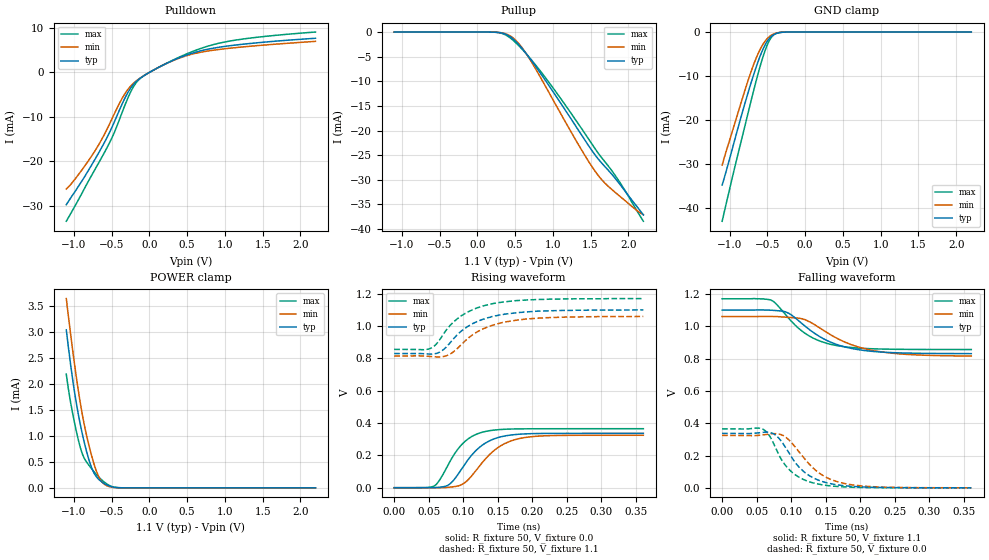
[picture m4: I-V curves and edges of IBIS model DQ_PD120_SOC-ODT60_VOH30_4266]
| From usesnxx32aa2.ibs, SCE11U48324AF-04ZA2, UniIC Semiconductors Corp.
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| DQ_PD120_SOC-ODT60_VOH30_4266
| (120 Ohm Pulldown, 60 Ohm System ODT Setting, VOH=VDDQ/3.0, 3200-4266Mbps)
[Model]   DQ_PD120_SOC-ODT60_VOH30_4266
Model_type   I/O
Vinl = 123.333mV
Vinh = 243.333mV
Vmeas = 183.333mV
Vref = 0.0mV
Cref = 0.0pF
Rref = 60.000Ohm
|   typ   min   max
|C_comp   0.797pF   0.747pF   0.847pF
C_comp_pullup   0.3985pF   0.3735pF   0.4235pF
C_comp_pulldown   0.3985pF   0.3735pF   0.4235pF
| Note: C_comp changes when the ODT circuit is enabled.
[Model Spec]
| Input threshold voltage corners
Vinl   0.1233V   0.1167V   0.1350V
Vinh   0.2433V   0.2367V   0.2550V
| Measurement voltage corners
Vmeas   0.1833V   0.1767V   0.1950V
| Timing spec test load voltage corners
Vref   0.0000V   0.0000V   0.0000V
| Dynamic Overshoot Parameters from LPDDR4 Specification
D_overshoot_ampl_h   0.30   NA   NA
D_overshoot_ampl_l   0.30   NA   NA
D_overshoot_area_h   0.1n   NA   NA
D_overshoot_area_l   0.1n   NA   NA
[Receiver Thresholds]
Vth   = 0.1833V
Vth_min  = 0.1800V
Vth_max  = 0.1866V
Vinh_ac  = 0.060V
Vinh_dc  = 0.060V
Vinl_ac  = -0.060V
Vinl_dc  = -0.060V
Tslew_ac = 5.000ns |Not specified, so set to high value
Threshold_sensitivity = 0.1667
Reference_supply Pullup_ref
[Voltage Range]   1.1000V   1.0600V   1.1700V
[Pullup Reference]   1.1000V   1.0600V   1.1700V
| Junction Temperature (Ambient temp is 35C typ 95C min -40C max)
[Temperature Range]   50.0   110.0   -40.0
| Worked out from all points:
|   slope of the pulldown table from 0 to 0.165 V, typ, clamps not added: 109 ohm
|   slope of the pullup table from 0 to 0.165 V, typ, clamps not added: 19.3 kohm
|   GND clamp passes 1 mA (typ) near -0.45 V on its own axis
|   POWER clamp passes 1 mA (typ) near -0.88 V on its own axis
|   rising waveform, R_fixture 50, V_fixture 0.0: 20-80 % time 39.7ps typ, 43.9ps min, 34.6ps max; typ from 0.001 V to 0.337 V
|   falling waveform, R_fixture 50, V_fixture 1.1: 20-80 % time 60.4ps typ, 70ps min, 51ps max; typ from 1.1 V to 0.831 V
|   rising waveform, R_fixture 50, V_fixture 1.1: 20-80 % time 53.1ps typ, 54.9ps min, 50.7ps max; typ from 0.83 V to 1.1 V
|   falling waveform, R_fixture 50, V_fixture 0.0: 20-80 % time 40.6ps typ, 46.3ps min, 36.1ps max; typ from 0.337 V to 0.001 V
[Pulldown]
|   Voltage   I(typ)   I(min)   I(max)
-1.1V     -29.81mA   -26.27mA   -33.53mA
-921.8mV  -25.21mA   -22.63mA   -28.15mA
-697.4mV  -18.91mA   -17.05mA   -21.18mA
-489.5mV  -12.15mA   -10.27mA   -14.52mA
-314.6mV  -5.506mA   -4.574mA   -7.019mA
-205.7mV  -2.636mA   -2.392mA   -3.114mA
-100.1mV  -1.074mA   -1.047mA   -1.09mA
154mV     1.398mA    1.387mA    1.403mA
391.6mV   3.252mA    3.172mA    3.388mA
850.3mV   5.453mA    4.993mA    6.257mA
1.309V    6.458mA    5.837mA    7.66mA
2.2V      7.677mA    6.979mA    9.076mA
[GND Clamp]
|   Voltage   I(typ)   I(min)   I(max)
-1.1V     -34.88mA   -30.34mA   -43.13mA
-941.6mV  -25.13mA   -21.34mA   -31.48mA
-789.8mV  -15.79mA   -12.83mA   -20.82mA
-717.2mV  -11.61mA   -9.055mA   -15.72mA
-661.1mV  -8.596mA   -6.455mA   -11.9mA
-588.5mV  -5.128mA   -3.689mA   -7.329mA
-522.5mV  -2.673mA   -1.907mA   -3.823mA
-466.4mV  -1.296mA   -942.9uA   -1.693mA
-413.6mV  -566.4uA   -417.7uA   -621.8uA
-350.9mV  -165.9uA   -125.8uA   -147.4uA
-261.8mV  -17.68uA   -15.49uA   -11.04uA
2.2V      0A         0A         0A
[Pullup]
|   Voltage   I(typ)   I(min)   I(max)
-1.1V     4.189uA    6.456uA    1.888uA
229.9mV   -30.39uA   -30.49uA   -31.09uA
335.5mV   -227.7uA   -189uA     -313.1uA
441.1mV   -997.2uA   -819.6uA   -1.249mA
556.6mV   -2.66mA    -2.461mA   -2.874mA
691.9mV   -5.249mA   -5.417mA   -5.187mA
965.8mV   -11.24mA   -12.72mA   -10.55mA
1.292V    -18.81mA   -21.61mA   -17.61mA
1.589V    -25.54mA   -28.86mA   -24.33mA
1.688V    -27.28mA   -30.64mA   -26.3mA
1.89V     -30.93mA   -33.36mA   -30.56mA
2.2V      -37.14mA   -37.09mA   -38.43mA
[POWER Clamp]
|   Voltage   I(typ)   I(min)   I(max)
-1.1V     3.036mA    3.636mA    2.186mA
-1.041V   2.347mA    2.931mA    1.626mA
-977.9mV  1.724mA    2.243mA    1.161mA
-908.6mV  1.178mA    1.583mA    748.3uA
-852.5mV  818.6uA    1.149mA    543.7uA
-779.9mV  447.9uA    701.7uA    396.3uA
-713.9mV  239.2uA    373.2uA    278.6uA
-654.5mV  142.7uA    170.4uA    185.9uA
-598.4mV  83.65uA    72.04uA    113.1uA
-486.2mV  16.76uA    10.18uA    20.93uA
-367.4mV  1.193uA    876.9nA    944.7nA
2.2V      0A         0A         0A
[Ramp]
|   typ   min   max
| 20% - 80%
dV/dt_r   201.88m/39.68p   194.63m/43.89p   218.98m/34.58p
dV/dt_f   161.61m/60.39p   146.51m/69.99p   188.44m/50.89p
| 25% - 75%
|dV/dt_r   168.23m/31.62p   162.19m/34.98p   182.48m/27.48p
|dV/dt_f   134.67m/48.07p   122.09m/55.73p   157.04m/40.43p
R_load = 50
[Rising Waveform]
R_fixture = 50
V_fixture = 0.0
|   Time   V(typ)   V(min)   V(max)
0s        626.1uV    550.8uV    451.5uV
57ps      761.2uV    -59.79uV   9.486mV
65ps      3.351mV    -97.64uV   43.16mV
77ps      13.79mV    2.578mV    133.1mV
101ps     137.8mV    27.55mV    281mV
116ps     219.8mV    93.53mV    325.4mV
131ps     273.7mV    173mV      347.5mV
157ps     317.8mV    266.4mV    361.4mV
190ps     333.5mV    311.4mV    364.9mV
361ps     337.1mV    324.9mV    365.4mV
[Falling Waveform]
R_fixture   = 50
V_fixture   = 1.1
V_fixture_min = 1.06
V_fixture_max = 1.17
|   Time   V(typ)   V(min)   V(max)
0s        1.1V       1.06V      1.17V
70ps      1.099V     1.061V     1.163V
77ps      1.097V     1.06V      1.144V
92ps      1.089V     1.056V     1.071V
120ps     1.001V     1.041V     956.8mV
137ps     947.6mV    1.001V     916.4mV
161ps     895mV      937.9mV    884.6mV
191ps     859.7mV    880.5mV    867mV
229ps     840.9mV    842.4mV    859.2mV
361ps     830.7mV    815.8mV    855.9mV
[Rising Waveform]
R_fixture   = 50
V_fixture   = 1.1
V_fixture_min = 1.06
V_fixture_max = 1.17
|   Time   V(typ)   V(min)   V(max)
0s        830.3mV    814.6mV    855.9mV
51ps      826.7mV    812.6mV    859.7mV
61ps      830.8mV    809.5mV    888.8mV
75ps      868.6mV    815.7mV    973.4mV
89ps      936.6mV    851.8mV    1.037V
105ps     993.5mV    917.3mV    1.084V
122ps     1.031V     968.4mV    1.115V
144ps     1.061V     1.007V     1.14V
211ps     1.093V     1.05V      1.165V
361ps     1.1V       1.06V      1.17V
[Falling Waveform]
R_fixture = 50
V_fixture = 0.0
|   Time   V(typ)   V(min)   V(max)
0s        337.2mV    325.1mV    365.5mV
56ps      342.4mV    326.2mV    368.1mV
74ps      335.8mV    335.5mV    280.1mV
85ps      293.1mV    330.3mV    181.9mV
98ps      207.5mV    291.5mV    109.8mV
114ps     117.6mV    209.4mV    60.1mV
134ps     58.06mV    114.6mV    28.64mV
160ps     23.85mV    48.12mV    11.15mV
196ps     7.381mV    14.93mV    3.294mV
361ps     736.2uV    730.6uV    485.7uV
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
